|Texas Instruments Incorporated
|ADS127L18 8-channel,simultaneous-sampling,512-kSPS,wideband 24-bit del-sig ADC
|ADS127L14 4-channel,simultaneous-sampling,512-kSPS,wideband 24-bit del-sig ADC
|ADS117L18 8-channel,simultaneous-sampling,512-kSPS,wideband 16-bit del-sig ADC
|ADS117L14 4-channel,simultaneous-sampling,512-kSPS,wideband 16-bit del-sig ADC
[IBIS Ver]   4.1
[File name]   ads127l14-8.ibs
[Date]   01/25/2025
[File Rev]   1.0
[Source]
| Texas Instruments Incorporated.
| 12500 TI Blvd
| Dallas, TX -75243
[Notes]   Revision History:
| Rev 1.0: 05/04/2024
| - Initial version of the model
| - Model generated from simulations in SPECTRE
| - C_comp although listed in numerical order of value are
|   obtained from varying PVT conditions. For PVT conditions for
|   each specific value refer the buffer description under
|   respective [Model]. IBIS model user is responsible for using
|   appropriate C_comp to simulate for Signal Integrity.
| - Warnings regarding combined Non-monotonicity of various models have been
|   reviewed and considered minor and can be ignored
[Disclaimer]
| This model is designed as an aid for customers of Texas Instruments.
| TI and its licensors and suppliers make no warranties, either expressed
| or implied, with respect to this  model, including the warranties of
| merchantability or fitness for a particular purpose. The model is
| provided solely on an "as is" basis. The entire risk as to its quality
| and performance is with the customer.
| This model is subject to change without notice. Texas Instruments
| Incorporated is not responsible for updating this model.
[Copyright]
(C) Copyright 2019 Texas Instruments Incorporated.All rights reserved.
| ADS127L18RSH 56-pin VQFN-RSH package
[Component] ADS127L18RSH
[Manufacturer] Texas Instruments Incorporated
[Package] |VQFN(RSH) 56-pin
|variable   typ   min   max
R_pkg   0.07   0.05   0.09
L_pkg   1.1nH   0.8nH   1.4nH
C_pkg   0.18pF   0.15pF   0.21pF
[Pin] signal_name   model_name   R_pin   L_pin   C_pin
1   SDI/OSR0   input   NA   NA   NA
2   SDO/OSR1   io   NA   NA   NA
3   GPIO0/TDM   io   NA   NA   NA
4   GPIO1/HDR   io   NA   NA   NA
5   ERRORn   output_errorn   NA   NA   NA
6   DOUT0   output_data   NA   NA   NA
7   DOUT1   output_data   NA   NA   NA
8   DOUT2/GPIO2   io   NA   NA   NA
9   DOUT3/GPIO3   io   NA   NA   NA
10   DOUT4/DIN3/GPIO4   io   NA   NA   NA
11   DOUT5/DIN2/GPIO5   io   NA   NA   NA
12   DOUT6/DIN1/GPIO6   io   NA   NA   NA
13   DOUT7/DIN0/GPIO7   io   NA   NA   NA
14   DCLK   output_dclk   NA   NA   NA
15   FSYNC   io   NA   NA   NA
16   CLKIN   input   NA   NA   NA
17   DGND   GND   NA   NA   NA
18   IOVDD   POWER   NA   NA   NA
19   IOVDD   POWER   NA   NA   NA
20   CAPD   NC   NA   NA   NA
21   DGND   GND   NA   NA   NA
22   AVSS   GND   NA   NA   NA
23   AVDD1   POWER   NA   NA   NA
24   AVDD1   POWER   NA   NA   NA
25   AVDD2   POWER   NA   NA   NA
26   CAPA   NC   NA   NA   NA
27   CAPA   NC   NA   NA   NA
28   AVSS   GND   NA   NA   NA
29   AINP7   NC   NA   NA   NA
30   AINN7   NC   NA   NA   NA
31   AINP6   NC   NA   NA   NA
32   AINN6   NC   NA   NA   NA
33   AINP5   NC   NA   NA   NA
34   AINN5   NC   NA   NA   NA
35   AINP4   NC   NA   NA   NA
36   AINN4   NC   NA   NA   NA
37   AINP3   NC   NA   NA   NA
38   AINN3   NC   NA   NA   NA
39   AINP2   NC   NA   NA   NA
40   AINN2   NC   NA   NA   NA
41   AINP1   NC   NA   NA   NA
42   AINN1   NC   NA   NA   NA
43   AINP0   NC   NA   NA   NA
44   AINN0   NC   NA   NA   NA
45   AVSS   GND   NA   NA   NA
46   VCM   NC   NA   NA   NA
47   REFN   NC   NA   NA   NA
48   REFN   NC   NA   NA   NA
49   REFP   NC   NA   NA   NA
50   REFP   NC   NA   NA   NA
51   AVSS   GND   NA   NA   NA
52   RESETn   input   NA   NA   NA
53   START   input   NA   NA   NA
54   MODE   input   NA   NA   NA
55   CSn/SPEED   input   NA   NA   NA
56   SCLK/FLTR   input   NA   NA   NA
|***** end of component definition
| ADS127L14RSH 56-pin VQFN-RSH package
[Component] ADS127L14RSH
[Manufacturer] Texas Instruments Incorporated
[Package] |VQFN(RSH) 56-pin
|variable   typ   min   max
R_pkg   0.07   0.05   0.09
L_pkg   1.1nH   0.8nH   1.4nH
C_pkg   0.18pF   0.15pF   0.21pF
[Pin] signal_name   model_name   R_pin   L_pin   C_pin
1   SDI/OSR0   input   NA   NA   NA
2   SDO/OSR1   io   NA   NA   NA
3   GPIO0/TDM   io   NA   NA   NA
4   GPIO1/HDR   io   NA   NA   NA
5   ERRORn   output_errorn   NA   NA   NA
6   DOUT0   output_data   NA   NA   NA
7   DOUT1   output_data   NA   NA   NA
8   DOUT2/GPIO2   io   NA   NA   NA
9   DOUT3/GPIO3   io   NA   NA   NA
10   DOUT4/DIN3/GPIO4   io   NA   NA   NA
11   DOUT5/DIN2/GPIO5   io   NA   NA   NA
12   DOUT6/DIN1/GPIO6   io   NA   NA   NA
13   DOUT7/DIN0/GPIO7   io   NA   NA   NA
14   DCLK   output_dclk   NA   NA   NA
15   FSYNC   io   NA   NA   NA
16   CLKIN   input   NA   NA   NA
17   DGND   GND   NA   NA   NA
18   IOVDD   POWER   NA   NA   NA
19   IOVDD   POWER   NA   NA   NA
20   CAPD   NC   NA   NA   NA
21   DGND   GND   NA   NA   NA
22   AVSS   GND   NA   NA   NA
23   AVDD1   POWER   NA   NA   NA
24   AVDD1   POWER   NA   NA   NA
25   AVDD2   POWER   NA   NA   NA
26   CAPA   NC   NA   NA   NA
27   CAPA   NC   NA   NA   NA
28   AVSS   GND   NA   NA   NA
29   AVSS   GND   NA   NA   NA
30   AVSS   GND   NA   NA   NA
31   AVSS   GND   NA   NA   NA
32   AVSS   GND   NA   NA   NA
33   AVSS   GND   NA   NA   NA
34   AVSS   GND   NA   NA   NA
35   AVSS   GND   NA   NA   NA
36   AVSS   GND   NA   NA   NA
37   AINP3   NC   NA   NA   NA
38   AINN3   NC   NA   NA   NA
39   AINP2   NC   NA   NA   NA
40   AINN2   NC   NA   NA   NA
41   AINP1   NC   NA   NA   NA
42   AINN1   NC   NA   NA   NA
43   AINP0   NC   NA   NA   NA
44   AINN0   NC   NA   NA   NA
45   AVSS   GND   NA   NA   NA
46   VCM   NC   NA   NA   NA
47   REFN   NC   NA   NA   NA
48   REFN   NC   NA   NA   NA
49   REFP   NC   NA   NA   NA
50   REFP   NC   NA   NA   NA
51   AVSS   GND   NA   NA   NA
52   RESETn   input   NA   NA   NA
53   START   input   NA   NA   NA
54   MODE   input   NA   NA   NA
55   CSn/SPEED   input   NA   NA   NA
56   SCLK/FLTR   input   NA   NA   NA
|***** end of component definition
| ADS117L18RSH 56-pin VQFN-RSH package
[Component] ADS117L18RSH
[Manufacturer] Texas Instruments Incorporated
[Package] |VQFN(RSH) 56-pin
|variable   typ   min   max
R_pkg   0.07   0.05   0.09
L_pkg   1.1nH   0.8nH   1.4nH
C_pkg   0.18pF   0.15pF   0.21pF
[Pin] signal_name   model_name   R_pin   L_pin   C_pin
1   SDI/OSR0   input   NA   NA   NA
2   SDO/OSR1   io   NA   NA   NA
3   GPIO0/TDM   io   NA   NA   NA
4   GPIO1/HDR   io   NA   NA   NA
5   ERRORn   output_errorn   NA   NA   NA
6   DOUT0   output_data   NA   NA   NA
7   DOUT1   output_data   NA   NA   NA
8   DOUT2/GPIO2   io   NA   NA   NA
9   DOUT3/GPIO3   io   NA   NA   NA
10   DOUT4/DIN3/GPIO4   io   NA   NA   NA
11   DOUT5/DIN2/GPIO5   io   NA   NA   NA
12   DOUT6/DIN1/GPIO6   io   NA   NA   NA
13   DOUT7/DIN0/GPIO7   io   NA   NA   NA
14   DCLK   output_dclk   NA   NA   NA
15   FSYNC   io   NA   NA   NA
16   CLKIN   input   NA   NA   NA
17   DGND   GND   NA   NA   NA
18   IOVDD   POWER   NA   NA   NA
19   IOVDD   POWER   NA   NA   NA
20   CAPD   NC   NA   NA   NA
21   DGND   GND   NA   NA   NA
22   AVSS   GND   NA   NA   NA
23   AVDD1   POWER   NA   NA   NA
24   AVDD1   POWER   NA   NA   NA
25   AVDD2   POWER   NA   NA   NA
26   CAPA   NC   NA   NA   NA
27   CAPA   NC   NA   NA   NA
28   AVSS   GND   NA   NA   NA
29   AINP7   NC   NA   NA   NA
30   AINN7   NC   NA   NA   NA
31   AINP6   NC   NA   NA   NA
32   AINN6   NC   NA   NA   NA
33   AINP5   NC   NA   NA   NA
34   AINN5   NC   NA   NA   NA
35   AINP4   NC   NA   NA   NA
36   AINN4   NC   NA   NA   NA
37   AINP3   NC   NA   NA   NA
38   AINN3   NC   NA   NA   NA
39   AINP2   NC   NA   NA   NA
40   AINN2   NC   NA   NA   NA
41   AINP1   NC   NA   NA   NA
42   AINN1   NC   NA   NA   NA
43   AINP0   NC   NA   NA   NA
44   AINN0   NC   NA   NA   NA
45   AVSS   GND   NA   NA   NA
46   VCM   NC   NA   NA   NA
47   REFN   NC   NA   NA   NA
48   REFN   NC   NA   NA   NA
49   REFP   NC   NA   NA   NA
50   REFP   NC   NA   NA   NA
51   AVSS   GND   NA   NA   NA
52   RESETn   input   NA   NA   NA
53   START   input   NA   NA   NA
54   MODE   input   NA   NA   NA
55   CSn/SPEED   input   NA   NA   NA
56   SCLK/FLTR   input   NA   NA   NA
|***** end of component definition
| ADS117L14RSH 56-pin VQFN-RSH package
[Component] ADS117L14RSH
[Manufacturer] Texas Instruments Incorporated
[Package] |VQFN(RSH) 56-pin
|variable   typ   min   max
R_pkg   0.07   0.05   0.09
L_pkg   1.1nH   0.8nH   1.4nH
C_pkg   0.18pF   0.15pF   0.21pF
[Pin] signal_name   model_name   R_pin   L_pin   C_pin
1   SDI/OSR0   input   NA   NA   NA
2   SDO/OSR1   io   NA   NA   NA
3   GPIO0/TDM   io   NA   NA   NA
4   GPIO1/HDR   io   NA   NA   NA
5   ERRORn   output_errorn   NA   NA   NA
6   DOUT0   output_data   NA   NA   NA
7   DOUT1   output_data   NA   NA   NA
8   DOUT2/GPIO2   io   NA   NA   NA
9   DOUT3/GPIO3   io   NA   NA   NA
10   DOUT4/DIN3/GPIO4   io   NA   NA   NA
11   DOUT5/DIN2/GPIO5   io   NA   NA   NA
12   DOUT6/DIN1/GPIO6   io   NA   NA   NA
13   DOUT7/DIN0/GPIO7   io   NA   NA   NA
14   DCLK   output_dclk   NA   NA   NA
15   FSYNC   io   NA   NA   NA
16   CLKIN   input   NA   NA   NA
17   DGND   GND   NA   NA   NA
18   IOVDD   POWER   NA   NA   NA
19   IOVDD   POWER   NA   NA   NA
20   CAPD   NC   NA   NA   NA
21   DGND   GND   NA   NA   NA
22   AVSS   GND   NA   NA   NA
23   AVDD1   POWER   NA   NA   NA
24   AVDD1   POWER   NA   NA   NA
25   AVDD2   POWER   NA   NA   NA
26   CAPA   NC   NA   NA   NA
27   CAPA   NC   NA   NA   NA
28   AVSS   GND   NA   NA   NA
29   AVSS   GND   NA   NA   NA
30   AVSS   GND   NA   NA   NA
31   AVSS   GND   NA   NA   NA
32   AVSS   GND   NA   NA   NA
33   AVSS   GND   NA   NA   NA
34   AVSS   GND   NA   NA   NA
35   AVSS   GND   NA   NA   NA
36   AVSS   GND   NA   NA   NA
37   AINP3   NC   NA   NA   NA
38   AINN3   NC   NA   NA   NA
39   AINP2   NC   NA   NA   NA
40   AINN2   NC   NA   NA   NA
41   AINP1   NC   NA   NA   NA
42   AINN1   NC   NA   NA   NA
43   AINP0   NC   NA   NA   NA
44   AINN0   NC   NA   NA   NA
45   AVSS   GND   NA   NA   NA
46   VCM   NC   NA   NA   NA
47   REFN   NC   NA   NA   NA
48   REFN   NC   NA   NA   NA
49   REFP   NC   NA   NA   NA
50   REFP   NC   NA   NA   NA
51   AVSS   GND   NA   NA   NA
52   RESETn   input   NA   NA   NA
53   START   input   NA   NA   NA
54   MODE   input   NA   NA   NA
55   CSn/SPEED   input   NA   NA   NA
56   SCLK/FLTR   input   NA   NA   NA
|***** end of component definition
[Model Selector] io
io_fp io buffer with user register field OUT_DRV = 0b
io_hp io buffer with user register field OUT_DRV = 1b
[Model Selector] output_errorn
output_errorn_fp output buffer with user register field OUT_DRV = 0b
output_errorn_hp output buffer with user register field OUT_DRV = 1b
[Model Selector] output_data
output_data_fp output buffer with user register field OUT_DRV = 0b
output_data_hp output buffer with user register field OUT_DRV = 1b
[Model Selector] output_dclk
output_dclk_fp output buffer with user register field OUT_DRV = 0b
output_dclk_hp output buffer with user register field OUT_DRV = 1b
| Models and submodels in the file (9): io_fp (I/O), io_hp (I/O), output_errorn_fp (Open_drain), output_errorn_hp (Open_drain), output_data_fp (Output), output_data_hp (Output), output_dclk_fp (Output), output_dclk_hp (Output), input (Input)
